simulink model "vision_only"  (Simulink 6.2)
settings: Solver=ode45  StartTime=0.0  StopTime=inf  RelTol=1e-3
libraries: xpclib x4, simulink x2

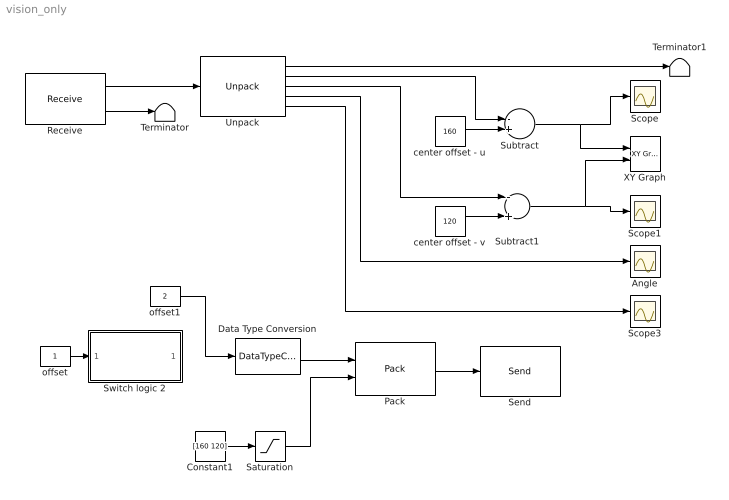
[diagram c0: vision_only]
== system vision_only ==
  Angle : Scope
  Constant1 : Constant  Value=[160 120]
  Data Type Conversion : DataTypeConversion  OutDataTypeMode=uint8
  Pack : xpclib/UDP/Pack  datatypes={'uint8','double'}  byteAlign=4
  Receive : xpclib/UDP/Receive  ipAddress=127.0.0.1  ipPort=6907  width=40  sampletime=h
  Saturation : Saturate  UpperLimit=[320 240]  LowerLimit=[0 0]
  Scope : Scope
  Scope1 : Scope
  Scope3 : Scope
  Send : xpclib/UDP/Send  ipAddress=127.0.0.1  ipPort=6906  localPort=-1  sampletime=h
  Subtract : Sum  Inputs=-+  OutScaling=2^-10
  Subtract1 : Sum  Inputs=-+  OutScaling=2^-10
  Switch logic 2 : Subsystem
  Terminator : Terminator
  Terminator1 : Terminator
  Unpack : xpclib/UDP/Unpack  dimensions={1,1,1,1,1}  datatypes={'double','double','double','double','double'}  byteAlign=4
  XY Graph : simulink/Sinks/XY Graph  xmin=-160  xmax=160  ymin=-120  ymax=120  st=-1
  center offset - u : Constant  Value=160
  center offset - v : Constant  Value=120
  offset : Constant
  offset1 : Constant  Value=2
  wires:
  Receive/2 -> Terminator/1
  Receive/1 -> Unpack/1
  Unpack/1 -> Terminator1/1
  center offset - u/1 -> Subtract/2
  center offset - v/1 -> Subtract1/2
  Unpack/2 -> Subtract/1
  Unpack/3 -> Subtract1/1
  Unpack/4 -> Angle/1
  Subtract/1 -> Scope/1, XY Graph/1
  Subtract1/1 -> Scope1/1, XY Graph/2
  Unpack/5 -> Scope3/1
  Pack/1 -> Send/1
  offset/1 -> Switch logic 2/1(In1)
  Constant1/1 -> Saturation/1
  Data Type Conversion/1 -> Pack/1
  Saturation/1 -> Pack/2
  offset1/1 -> Data Type Conversion/1

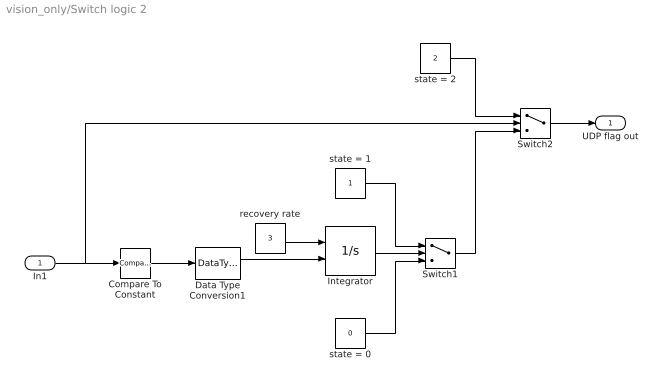
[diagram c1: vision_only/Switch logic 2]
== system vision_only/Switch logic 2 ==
  In1 : Inport  Port=1  LatchInput=off
  Compare To Constant : simulink/Logic and Bit Operations/Compare To Constant  relop=<  const=1  LogicOutDataTypeMode=uint8  ZeroCross=off
  Data Type Conversion1 : DataTypeConversion  OutDataTypeMode=boolean
  Integrator : Integrator  ExternalReset=rising  LimitOutput=on  UpperSaturationLimit=1  LowerSaturationLimit=0
  Switch1 : Switch  Threshold=0.5
  Switch2 : Switch  Threshold=1
  recovery rate : Constant  Value=3
  state = 0 : Constant  Value=0
  state = 1 : Constant
  state = 2 : Constant  Value=2
  UDP flag out : Outport
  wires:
  state = 1/1 -> Switch1/1
  state = 0/1 -> Switch1/3
  Integrator/1 -> Switch1/2
  Data Type Conversion1/1 -> Integrator/2
  recovery rate/1 -> Integrator/1
  state = 2/1 -> Switch2/1
  Compare To Constant/1 -> Data Type Conversion1/1
  Switch1/1 -> Switch2/3
  Switch2/1 -> UDP flag out/1
  In1/1 -> Compare To Constant/1, Switch2/2
